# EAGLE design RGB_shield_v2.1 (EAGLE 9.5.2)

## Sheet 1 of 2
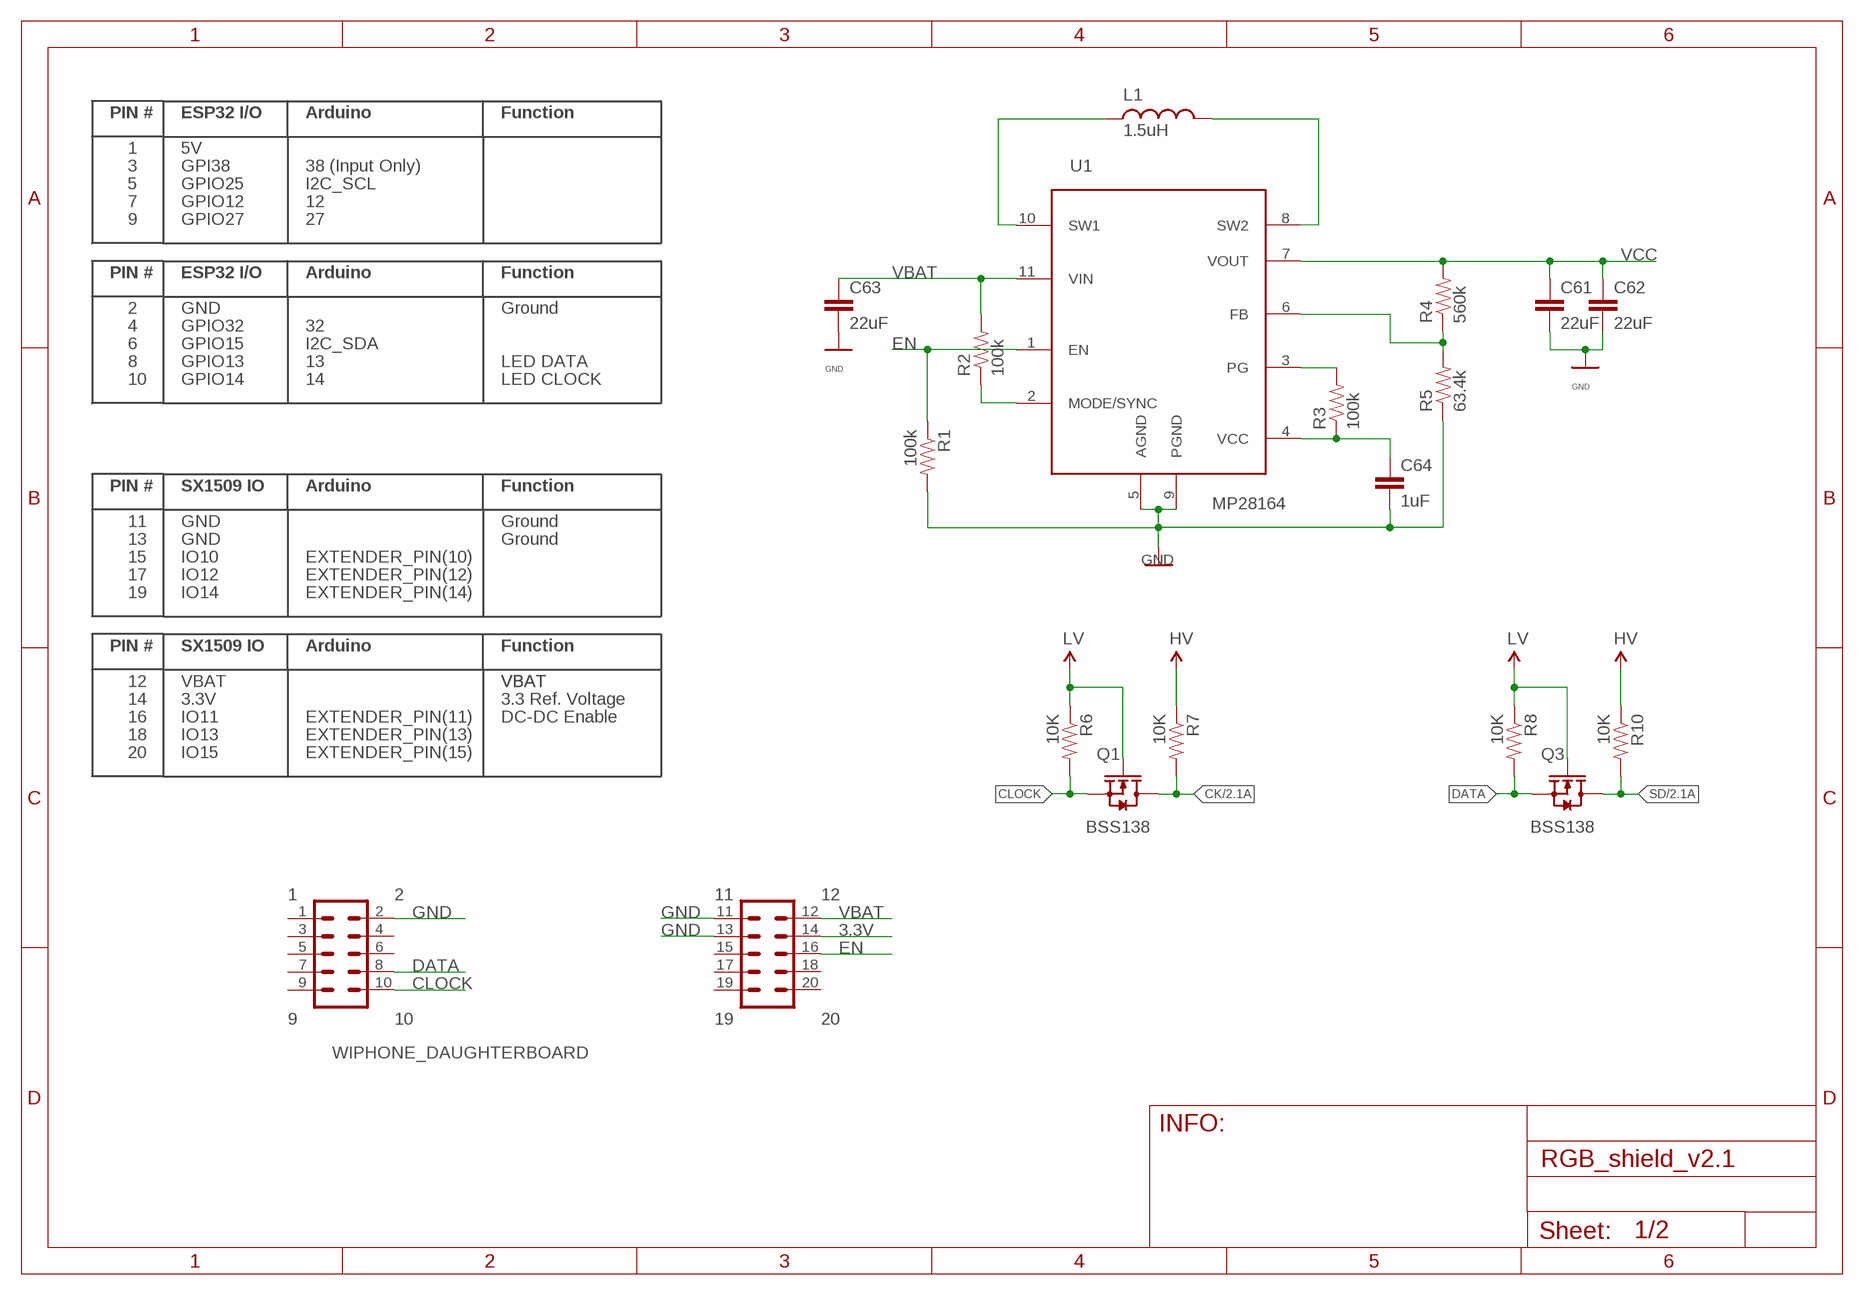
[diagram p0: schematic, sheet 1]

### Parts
C61  22uF  CAP  [0603-CAP-L]
C62  22uF  CAP  [0603-CAP-L]
C63  22uF  CAP0805  [0805_CAP]
C64  1uF  CAP  [0603-CAP-L]
L1  1.5uH  IND0420  [IND04020]
Q1  BSS138  MOSFET_N-L  [SOT23-3-L]
Q3  BSS138  MOSFET_N-L  [SOT23-3-L]
R1  100k  RES  [0603-RES-L]
R2  100k  RES  [0603-RES-L]
R3  100k  RES  [0603-RES-L]
R4  560k  RES  [0603-RES-L]
R5  63.4k  RES  [0603-RES-L]
R6  10K  RES0603  [0603-RES]
R7  10K  RES0603  [0603-RES]
R8  10K  RES0603  [0603-RES]
R10  10K  RES0603  [0603-RES]
U1  MP28164  [QFN11(MP28164)]
WIPHONE_DAUGHTERBOARD-FOOTPRINT1  WIPHONE_DAUGHTERBOARD  [WIPHONE_DAUGHTERBOARD]

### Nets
3.3V: Q1.1(G) Q3.1(G) R6.1 R8.1 WIPHONE_DAUGHTERBOARD-FOOTPRINT1.14 ; supply symbol labelled LV
CK: Q1.3(D) R7.2 ; also sheet 2
CLOCK: Q1.2(S) R6.2 WIPHONE_DAUGHTERBOARD-FOOTPRINT1.10
DATA: Q3.2(S) R8.2 WIPHONE_DAUGHTERBOARD-FOOTPRINT1.8
EN: R1.1 U1.1(EN) WIPHONE_DAUGHTERBOARD-FOOTPRINT1.16
GND: C61.2 C62.2 C63.2 C64.2 R1.2 R5.1 U1.5(AGND) U1.9(PGND) WIPHONE_DAUGHTERBOARD-FOOTPRINT1.2 WIPHONE_DAUGHTERBOARD-FOOTPRINT1.11 WIPHONE_DAUGHTERBOARD-FOOTPRINT1.13 ; also sheet 2
N$157: R2.1 U1.2(MODE/SYNC)
N$158: R3.2 U1.3(PG)
N$159: C64.1 R3.1 U1.4(VCC)
N$162: R4.1 R5.2 U1.6(FB)
SD: Q3.3(D) R10.2 ; also sheet 2
SW1: L1.1 U1.10(SW1)
SW2: L1.2 U1.8(SW2)
VBAT: C63.1 R2.2 U1.11(VIN) WIPHONE_DAUGHTERBOARD-FOOTPRINT1.12
VCC: C61.1 C62.1 R4.2 R7.1 R10.1 U1.7(VOUT) ; supply symbol labelled HV ; also sheet 2
Unconnected: WIPHONE_DAUGHTERBOARD-FOOTPRINT1.3 WIPHONE_DAUGHTERBOARD-FOOTPRINT1.4 WIPHONE_DAUGHTERBOARD-FOOTPRINT1.5 WIPHONE_DAUGHTERBOARD-FOOTPRINT1.6 WIPHONE_DAUGHTERBOARD-FOOTPRINT1.7 WIPHONE_DAUGHTERBOARD-FOOTPRINT1.9 WIPHONE_DAUGHTERBOARD-FOOTPRINT1.15 WIPHONE_DAUGHTERBOARD-FOOTPRINT1.17 WIPHONE_DAUGHTERBOARD-FOOTPRINT1.18 WIPHONE_DAUGHTERBOARD-FOOTPRINT1.19 WIPHONE_DAUGHTERBOARD-FOOTPRINT1.20

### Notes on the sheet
- Ground
- LED DATA
- LED CLOCK
- Ground
- Ground
- VBAT | VBAT
- 3.3 Ref. Voltage
- DC-DC Enable

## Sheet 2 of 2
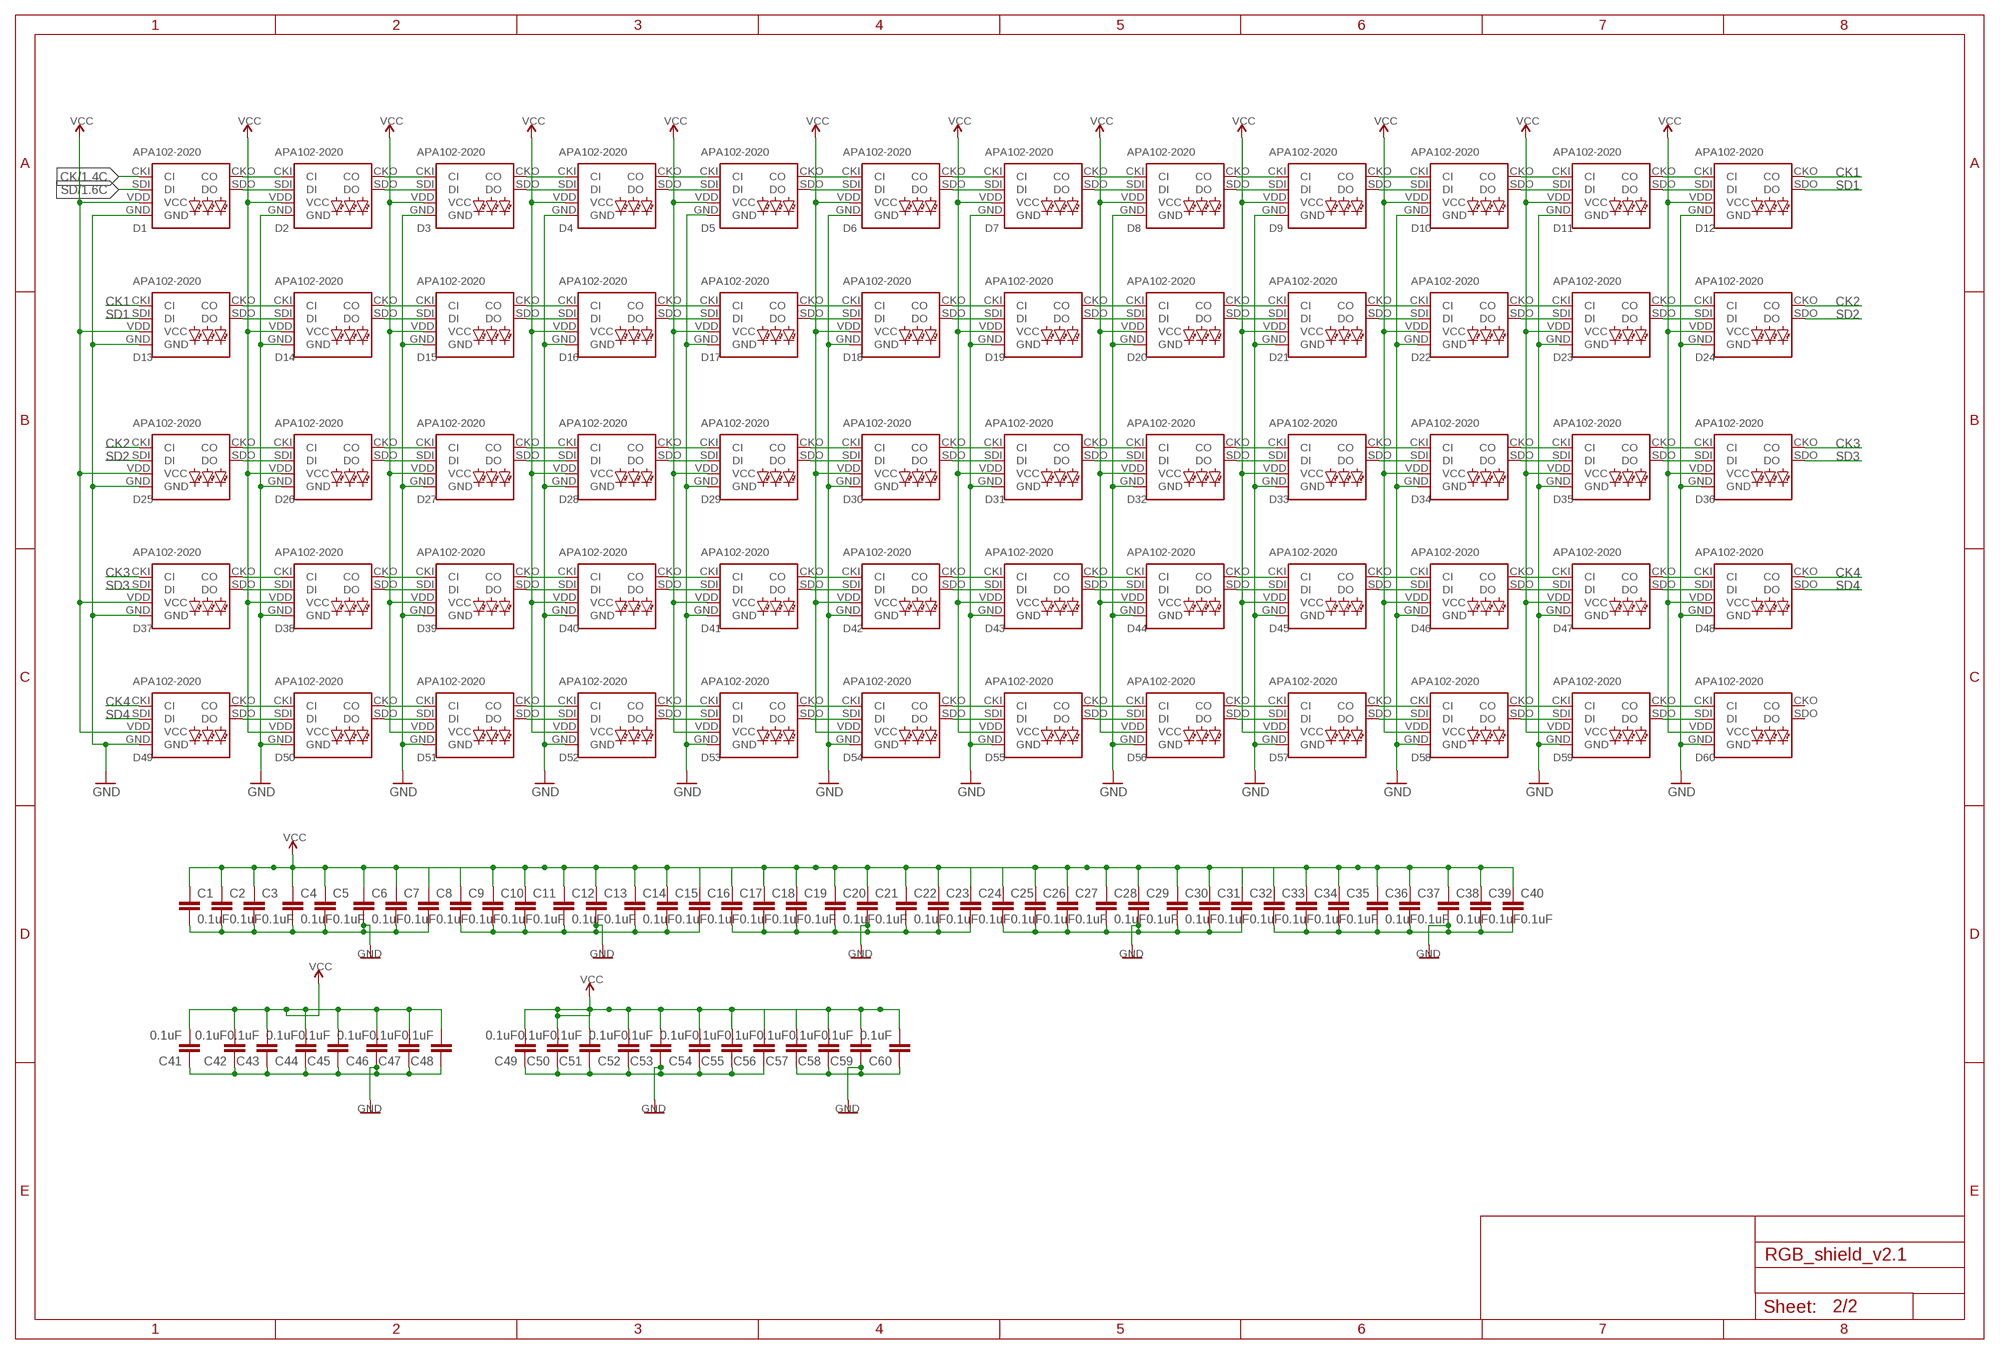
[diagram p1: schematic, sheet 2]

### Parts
C1  0.1uF  CAP0402  [0402-CAP]
C2  0.1uF  CAP0402  [0402-CAP]
C3  0.1uF  CAP0402  [0402-CAP]
C4  0.1uF  CAP0402  [0402-CAP]
C5  0.1uF  CAP0402  [0402-CAP]
C6  0.1uF  CAP0402  [0402-CAP]
C7  0.1uF  CAP0402  [0402-CAP]
C8  0.1uF  CAP0402  [0402-CAP]
C9  0.1uF  CAP0402  [0402-CAP]
C10  0.1uF  CAP0402  [0402-CAP]
C11  0.1uF  CAP0402  [0402-CAP]
C12  0.1uF  CAP0402  [0402-CAP]
C13  0.1uF  CAP0402  [0402-CAP]
C14  0.1uF  CAP0402  [0402-CAP]
C15  0.1uF  CAP0402  [0402-CAP]
C16  0.1uF  CAP0402  [0402-CAP]
C17  0.1uF  CAP0402  [0402-CAP]
C18  0.1uF  CAP0402  [0402-CAP]
C19  0.1uF  CAP0402  [0402-CAP]
C20  0.1uF  CAP0402  [0402-CAP]
C21  0.1uF  CAP0402  [0402-CAP]
C22  0.1uF  CAP0402  [0402-CAP]
C23  0.1uF  CAP0402  [0402-CAP]
C24  0.1uF  CAP0402  [0402-CAP]
C25  0.1uF  CAP0402  [0402-CAP]
C26  0.1uF  CAP0402  [0402-CAP]
C27  0.1uF  CAP0402  [0402-CAP]
C28  0.1uF  CAP0402  [0402-CAP]
C29  0.1uF  CAP0402  [0402-CAP]
C30  0.1uF  CAP0402  [0402-CAP]
C31  0.1uF  CAP0402  [0402-CAP]
C32  0.1uF  CAP0402  [0402-CAP]
C33  0.1uF  CAP0402  [0402-CAP]
C34  0.1uF  CAP0402  [0402-CAP]
C35  0.1uF  CAP0402  [0402-CAP]
C36  0.1uF  CAP0402  [0402-CAP]
C37  0.1uF  CAP0402  [0402-CAP]
C38  0.1uF  CAP0402  [0402-CAP]
C39  0.1uF  CAP0402  [0402-CAP]
C40  0.1uF  CAP0402  [0402-CAP]
C41  0.1uF  CAP0402  [0402-CAP]
C42  0.1uF  CAP0402  [0402-CAP]
C43  0.1uF  CAP0402  [0402-CAP]
C44  0.1uF  CAP0402  [0402-CAP]
C45  0.1uF  CAP0402  [0402-CAP]
C46  0.1uF  CAP0402  [0402-CAP]
C47  0.1uF  CAP0402  [0402-CAP]
C48  0.1uF  CAP0402  [0402-CAP]
C49  0.1uF  CAP0402  [0402-CAP]
C50  0.1uF  CAP0402  [0402-CAP]
C51  0.1uF  CAP0402  [0402-CAP]
C52  0.1uF  CAP0402  [0402-CAP]
C53  0.1uF  CAP0402  [0402-CAP]
C54  0.1uF  CAP0402  [0402-CAP]
C55  0.1uF  CAP0402  [0402-CAP]
C56  0.1uF  CAP0402  [0402-CAP]
C57  0.1uF  CAP0402  [0402-CAP]
C58  0.1uF  CAP0402  [0402-CAP]
C59  0.1uF  CAP0402  [0402-CAP]
C60  0.1uF  CAP0402  [0402-CAP]
D1  APA102-2020  [APA102-2020]
D2  APA102-2020  [APA102-2020]
D3  APA102-2020  [APA102-2020]
D4  APA102-2020  [APA102-2020]
D5  APA102-2020  [APA102-2020]
D6  APA102-2020  [APA102-2020]
D7  APA102-2020  [APA102-2020]
D8  APA102-2020  [APA102-2020]
D9  APA102-2020  [APA102-2020]
D10  APA102-2020  [APA102-2020]
D11  APA102-2020  [APA102-2020]
D12  APA102-2020  [APA102-2020]
D13  APA102-2020  [APA102-2020]
D14  APA102-2020  [APA102-2020]
D15  APA102-2020  [APA102-2020]
D16  APA102-2020  [APA102-2020]
D17  APA102-2020  [APA102-2020]
D18  APA102-2020  [APA102-2020]
D19  APA102-2020  [APA102-2020]
D20  APA102-2020  [APA102-2020]
D21  APA102-2020  [APA102-2020]
D22  APA102-2020  [APA102-2020]
D23  APA102-2020  [APA102-2020]
D24  APA102-2020  [APA102-2020]
D25  APA102-2020  [APA102-2020]
D26  APA102-2020  [APA102-2020]
D27  APA102-2020  [APA102-2020]
D28  APA102-2020  [APA102-2020]
D29  APA102-2020  [APA102-2020]
D30  APA102-2020  [APA102-2020]
D31  APA102-2020  [APA102-2020]
D32  APA102-2020  [APA102-2020]
D33  APA102-2020  [APA102-2020]
D34  APA102-2020  [APA102-2020]
D35  APA102-2020  [APA102-2020]
D36  APA102-2020  [APA102-2020]
D37  APA102-2020  [APA102-2020]
D38  APA102-2020  [APA102-2020]
D39  APA102-2020  [APA102-2020]
D40  APA102-2020  [APA102-2020]
D41  APA102-2020  [APA102-2020]
D42  APA102-2020  [APA102-2020]
D43  APA102-2020  [APA102-2020]
D44  APA102-2020  [APA102-2020]
D45  APA102-2020  [APA102-2020]
D46  APA102-2020  [APA102-2020]
D47  APA102-2020  [APA102-2020]
D48  APA102-2020  [APA102-2020]
D49  APA102-2020  [APA102-2020]
D50  APA102-2020  [APA102-2020]
D51  APA102-2020  [APA102-2020]
D52  APA102-2020  [APA102-2020]
D53  APA102-2020  [APA102-2020]
D54  APA102-2020  [APA102-2020]
D55  APA102-2020  [APA102-2020]
D56  APA102-2020  [APA102-2020]
D57  APA102-2020  [APA102-2020]
D58  APA102-2020  [APA102-2020]
D59  APA102-2020  [APA102-2020]
D60  APA102-2020  [APA102-2020]

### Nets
CK: D1.CKI(CI) ; also sheet 1
CK1: D12.CKO(CO) D13.CKI(CI)
CK2: D24.CKO(CO) D25.CKI(CI)
CK3: D36.CKO(CO) D37.CKI(CI)
CK4: D48.CKO(CO) D49.CKI(CI)
GND: C1.2 C2.2 C3.2 C4.2 C5.2 C6.2 C7.2 C8.2 C9.2 C10.2 C11.2 C12.2 C13.2 C14.2 C15.2 C16.2 C17.2 C18.2 C19.2 C20.2 C21.2 C22.2 C23.2 C24.2 C25.2 C26.2 C27.2 C28.2 C29.2 C30.2 C31.2 C32.2 C33.2 C34.2 C35.2 C36.2 C37.2 C38.2 C39.2 C40.2 C41.1 C42.1 C43.1 C44.1 C45.1 C46.1 C47.1 C48.1 C49.1 C50.1 C51.1 C52.1 C53.1 C54.1 C55.1 C56.1 C57.1 C58.1 C59.1 C60.1 D1.GND D2.GND D3.GND D4.GND D5.GND D6.GND D7.GND D8.GND D9.GND D10.GND D11.GND D12.GND D13.GND D14.GND D15.GND D16.GND D17.GND D18.GND D19.GND D20.GND D21.GND D22.GND D23.GND D24.GND D25.GND D26.GND D27.GND D28.GND D29.GND D30.GND D31.GND D32.GND D33.GND D34.GND D35.GND D36.GND D37.GND D38.GND D39.GND D40.GND D41.GND D42.GND D43.GND D44.GND D45.GND D46.GND D47.GND D48.GND D49.GND D50.GND D51.GND D52.GND D53.GND D54.GND D55.GND D56.GND D57.GND D58.GND D59.GND D60.GND ; also sheet 1
N$1: D1.CKO(CO) D2.CKI(CI)
N$2: D1.SDO(DO) D2.SDI(DI)
N$3: D2.CKO(CO) D3.CKI(CI)
N$4: D2.SDO(DO) D3.SDI(DI)
N$5: D3.CKO(CO) D4.CKI(CI)
N$6: D3.SDO(DO) D4.SDI(DI)
N$7: D4.CKO(CO) D5.CKI(CI)
N$8: D4.SDO(DO) D5.SDI(DI)
N$11: D5.CKO(CO) D6.CKI(CI)
N$12: D5.SDO(DO) D6.SDI(DI)
N$13: D6.CKO(CO) D7.CKI(CI)
N$14: D6.SDO(DO) D7.SDI(DI)
N$15: D7.CKO(CO) D8.CKI(CI)
N$16: D7.SDO(DO) D8.SDI(DI)
N$17: D8.CKO(CO) D9.CKI(CI)
N$18: D8.SDO(DO) D9.SDI(DI)
N$19: D9.CKO(CO) D10.CKI(CI)
N$20: D9.SDO(DO) D10.SDI(DI)
N$21: D10.CKO(CO) D11.CKI(CI)
N$22: D10.SDO(DO) D11.SDI(DI)
N$23: D11.CKO(CO) D12.CKI(CI)
N$24: D11.SDO(DO) D12.SDI(DI)
N$25: D13.CKO(CO) D14.CKI(CI)
N$26: D13.SDO(DO) D14.SDI(DI)
N$27: D14.CKO(CO) D15.CKI(CI)
N$28: D14.SDO(DO) D15.SDI(DI)
N$29: D15.CKO(CO) D16.CKI(CI)
N$30: D15.SDO(DO) D16.SDI(DI)
N$31: D16.CKO(CO) D17.CKI(CI)
N$32: D16.SDO(DO) D17.SDI(DI)
N$33: D17.CKO(CO) D18.CKI(CI)
N$34: D17.SDO(DO) D18.SDI(DI)
N$35: D18.CKO(CO) D19.CKI(CI)
N$36: D18.SDO(DO) D19.SDI(DI)
N$38: D19.CKO(CO) D20.CKI(CI)
N$40: D19.SDO(DO) D20.SDI(DI)
N$42: D20.CKO(CO) D21.CKI(CI)
N$43: D20.SDO(DO) D21.SDI(DI)
N$45: D21.CKO(CO) D22.CKI(CI)
N$47: D21.SDO(DO) D22.SDI(DI)
N$49: D22.CKO(CO) D23.CKI(CI)
N$50: D22.SDO(DO) D23.SDI(DI)
N$51: D23.CKO(CO) D24.CKI(CI)
N$52: D23.SDO(DO) D24.SDI(DI)
N$53: D25.CKO(CO) D26.CKI(CI)
N$54: D25.SDO(DO) D26.SDI(DI)
N$55: D26.CKO(CO) D27.CKI(CI)
N$56: D26.SDO(DO) D27.SDI(DI)
N$57: D27.CKO(CO) D28.CKI(CI)
N$58: D27.SDO(DO) D28.SDI(DI)
N$59: D28.CKO(CO) D29.CKI(CI)
N$60: D28.SDO(DO) D29.SDI(DI)
N$61: D29.CKO(CO) D30.CKI(CI)
N$62: D29.SDO(DO) D30.SDI(DI)
N$63: D30.CKO(CO) D31.CKI(CI)
N$64: D30.SDO(DO) D31.SDI(DI)
N$66: D31.CKO(CO) D32.CKI(CI)
N$67: D31.SDO(DO) D32.SDI(DI)
N$68: D32.CKO(CO) D33.CKI(CI)
N$69: D32.SDO(DO) D33.SDI(DI)
N$70: D33.CKO(CO) D34.CKI(CI)
N$72: D33.SDO(DO) D34.SDI(DI)
N$73: D34.CKO(CO) D35.CKI(CI)
N$74: D34.SDO(DO) D35.SDI(DI)
N$75: D35.CKO(CO) D36.CKI(CI)
N$77: D35.SDO(DO) D36.SDI(DI)
N$79: D37.CKO(CO) D38.CKI(CI)
N$81: D37.SDO(DO) D38.SDI(DI)
N$82: D38.CKO(CO) D39.CKI(CI)
N$91: D38.SDO(DO) D39.SDI(DI)
N$102: D39.CKO(CO) D40.CKI(CI)
N$103: D39.SDO(DO) D40.SDI(DI)
N$104: D40.CKO(CO) D41.CKI(CI)
N$105: D40.SDO(DO) D41.SDI(DI)
N$106: D41.CKO(CO) D42.CKI(CI)
N$107: D41.SDO(DO) D42.SDI(DI)
N$108: D42.CKO(CO) D43.CKI(CI)
N$109: D42.SDO(DO) D43.SDI(DI)
N$110: D43.CKO(CO) D44.CKI(CI)
N$111: D43.SDO(DO) D44.SDI(DI)
N$112: D44.CKO(CO) D45.CKI(CI)
N$113: D44.SDO(DO) D45.SDI(DI)
N$114: D45.CKO(CO) D46.CKI(CI)
N$115: D45.SDO(DO) D46.SDI(DI)
N$116: D46.CKO(CO) D47.CKI(CI)
N$117: D46.SDO(DO) D47.SDI(DI)
N$118: D47.CKO(CO) D48.CKI(CI)
N$119: D47.SDO(DO) D48.SDI(DI)
N$120: D49.CKO(CO) D50.CKI(CI)
N$121: D49.SDO(DO) D50.SDI(DI)
N$122: D50.CKO(CO) D51.CKI(CI)
N$123: D50.SDO(DO) D51.SDI(DI)
N$124: D51.CKO(CO) D52.CKI(CI)
N$125: D51.SDO(DO) D52.SDI(DI)
N$126: D52.CKO(CO) D53.CKI(CI)
N$127: D52.SDO(DO) D53.SDI(DI)
N$128: D53.CKO(CO) D54.CKI(CI)
N$129: D53.SDO(DO) D54.SDI(DI)
N$130: D54.CKO(CO) D55.CKI(CI)
N$131: D54.SDO(DO) D55.SDI(DI)
N$132: D55.CKO(CO) D56.CKI(CI)
N$133: D55.SDO(DO) D56.SDI(DI)
N$134: D57.CKO(CO) D58.CKI(CI)
N$135: D57.SDO(DO) D58.SDI(DI)
N$136: D58.CKO(CO) D59.CKI(CI)
N$137: D58.SDO(DO) D59.SDI(DI)
N$138: D59.CKO(CO) D60.CKI(CI)
N$139: D59.SDO(DO) D60.SDI(DI)
N$140: D56.CKO(CO) D57.CKI(CI)
N$141: D56.SDO(DO) D57.SDI(DI)
SD: D1.SDI(DI) ; also sheet 1
SD1: D12.SDO(DO) D13.SDI(DI)
SD2: D24.SDO(DO) D25.SDI(DI)
SD3: D36.SDO(DO) D37.SDI(DI)
SD4: D48.SDO(DO) D49.SDI(DI)
VCC: C1.1 C2.1 C3.1 C4.1 C5.1 C6.1 C7.1 C8.1 C9.1 C10.1 C11.1 C12.1 C13.1 C14.1 C15.1 C16.1 C17.1 C18.1 C19.1 C20.1 C21.1 C22.1 C23.1 C24.1 C25.1 C26.1 C27.1 C28.1 C29.1 C30.1 C31.1 C32.1 C33.1 C34.1 C35.1 C36.1 C37.1 C38.1 C39.1 C40.1 C41.2 C42.2 C43.2 C44.2 C45.2 C46.2 C47.2 C48.2 C49.2 C50.2 C51.2 C52.2 C53.2 C54.2 C55.2 C56.2 C57.2 C58.2 C59.2 C60.2 D1.VDD(VCC) D2.VDD(VCC) D3.VDD(VCC) D4.VDD(VCC) D5.VDD(VCC) D6.VDD(VCC) D7.VDD(VCC) D8.VDD(VCC) D9.VDD(VCC) D10.VDD(VCC) D11.VDD(VCC) D12.VDD(VCC) D13.VDD(VCC) D14.VDD(VCC) D15.VDD(VCC) D16.VDD(VCC) D17.VDD(VCC) D18.VDD(VCC) D19.VDD(VCC) D20.VDD(VCC) D21.VDD(VCC) D22.VDD(VCC) D23.VDD(VCC) D24.VDD(VCC) D25.VDD(VCC) D26.VDD(VCC) D27.VDD(VCC) D28.VDD(VCC) D29.VDD(VCC) D30.VDD(VCC) D31.VDD(VCC) D32.VDD(VCC) D33.VDD(VCC) D34.VDD(VCC) D35.VDD(VCC) D36.VDD(VCC) D37.VDD(VCC) D38.VDD(VCC) D39.VDD(VCC) D40.VDD(VCC) D41.VDD(VCC) D42.VDD(VCC) D43.VDD(VCC) D44.VDD(VCC) D45.VDD(VCC) D46.VDD(VCC) D47.VDD(VCC) D48.VDD(VCC) D49.VDD(VCC) D50.VDD(VCC) D51.VDD(VCC) D52.VDD(VCC) D53.VDD(VCC) D54.VDD(VCC) D55.VDD(VCC) D56.VDD(VCC) D57.VDD(VCC) D58.VDD(VCC) D59.VDD(VCC) D60.VDD(VCC) ; also sheet 1
Unconnected: D60.CKO(CO) D60.SDO(DO)

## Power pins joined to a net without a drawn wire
1: WIPHONE_DAUGHTERBOARD-FOOTPRINT1.1

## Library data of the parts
C1-C64 = WiPhone:CAP: Capacitor.
D1-D60 = WiPhone:APA102: APA102 Addressable RGB LED Used in manufacturing of various products at SparkFun Packages: 5050 2020 SparkFun Products: SparkFun Lumenati Boards; PROD_ID: DIO-13883
L1 = WiPhone:IND: Inductor.
Q1 Q3 = WiPhone:MOSFET_N: N-Channel Mosfet
R1-R8 R10 = WiPhone:RES: Resistor.
U1 = WiPhone:MP28164
WIPHONE_DAUGHTERBOARD-FOOTPRINT1 = WiPhone:WIPHONE_DAUGHTERBOARD

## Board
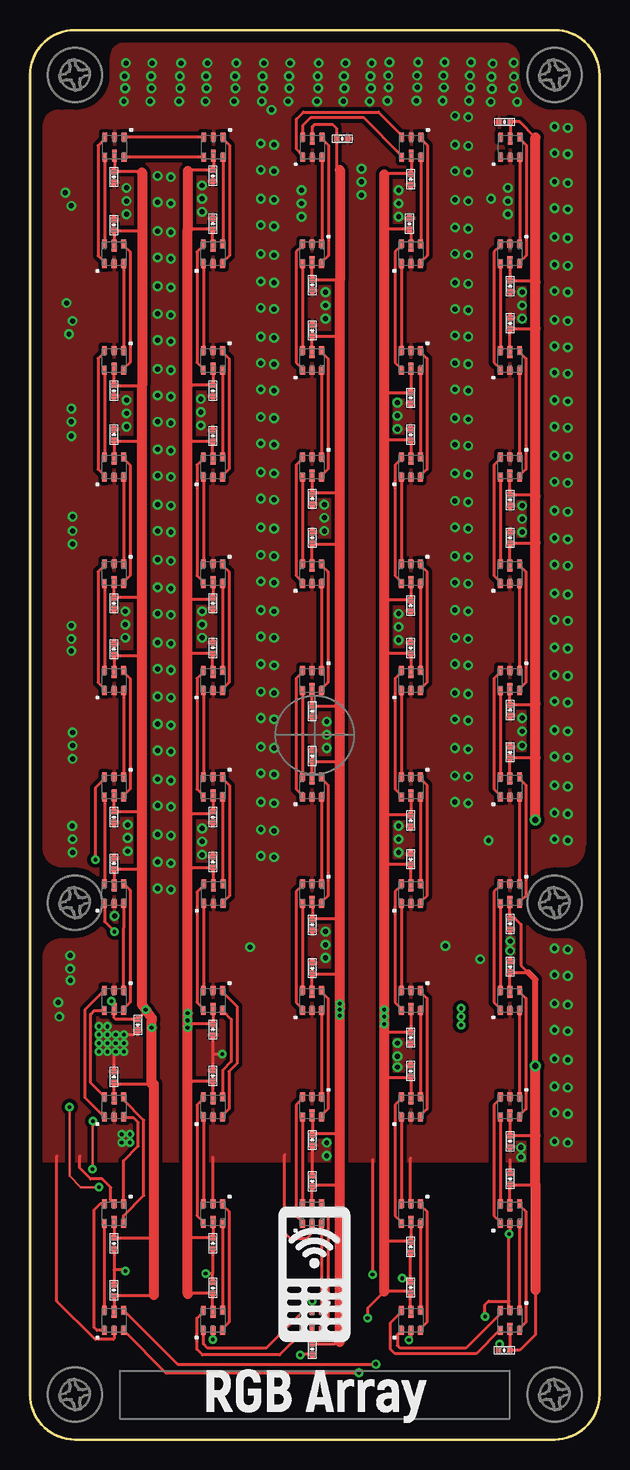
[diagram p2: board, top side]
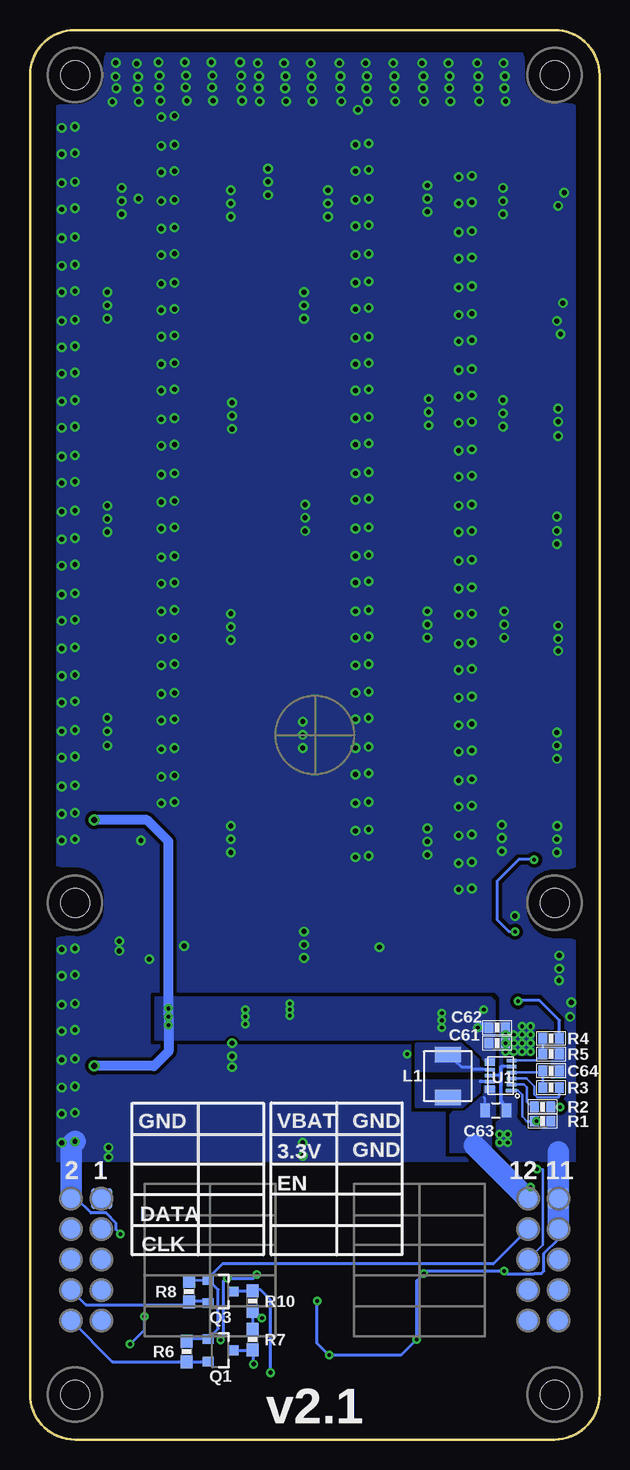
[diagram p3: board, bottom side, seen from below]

Size 47.5 x 117.5 mm. Coordinates in mm from the lower left corner, seen from the top.
Copper layers (1*16): Top 0.035mm / dielectric 1.5mm / Bottom 0.035mm
Design rules "2LDaughterBoards *": minimum track width 6mil, minimum drill 0.3mm, track to track 8mil, track to pad 8mil, pad to pad 8mil, via to via 8mil, smd to smd 0mil, copper to edge 16mil, drill to drill 6mil, minimum pad ring 10mil, minimum via ring 8mil, stop-mask expansion 4mil, vias tented up to drill 25mil, thermal gap 10mil

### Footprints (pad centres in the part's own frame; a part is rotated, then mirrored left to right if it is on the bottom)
0402-CAP = smd 0.508 x 0.508: 1 -0.457,0; 2 0.457,0
0603-CAP-L = smd 0.75 x 0.9: 1 -0.7,0; 2 0.7,0
0805_CAP = smd 0.8 x 1.2: 1 -0.9,0; 2 0.9,0
APA102-2020 = smd 0.4 x 0.7: CKI -0.8,-0.85; CKO 0.8,-0.85; GND 0,0.85; SDI -0.8,0.85; SDO 0.8,0.85 | smd 0.4 x 1: VDD 0,-0.7
IND04020 = smd 1.295 x 2.184: 1 -1.85,0; 2 1.748,0
SOT23-3-L = smd 0.8 x 0.9: 1 -0.95,-1; 2 0.95,-1; 3 0,1.1
0603-RES-L = smd 0.75 x 0.9: 1 -0.7,0; 2 0.7,0
0603-RES = smd 1.1 x 1: 1 -0.85,0; 2 0.85,0
QFN11(MP28164) = smd 0.9 x 0.3: 1 -0.9,1.25 | smd 0.8 x 0.3: 2 -0.9,0.75; 3 -0.9,0.25; 4 -0.9,-0.25; 5 -0.9,-0.75; 6 -0.9,-1.25; 8 0.9,-0.5; 9 0.9,0; 10 0.9,0.5 | smd 0.8 x 0.6: 7 0.9,-1.125; 11 0.9,1.125
WIPHONE_DAUGHTERBOARD = smd 1.75 x 1.75 bottom: 1 17.78,-38.66; 2 20.32,-38.66; 3 17.78,-41.2; 4 20.32,-41.2; 5 17.78,-43.74; 6 20.32,-43.74; 7 17.78,-46.28; 8 20.32,-46.28; 9 17.78,-48.82; 10 20.32,-48.82; 11 -20.32,-38.66; 12 -17.78,-38.66; 13 -20.32,-41.2; 14 -17.78,-41.2; 15 -20.32,-43.74; 16 -17.78,-43.74; 17 -20.32,-46.28; 18 -17.78,-46.28; 19 -20.32,-48.82; 20 -17.78,-48.82 | hole 2.4: 20,-54.991; -20,-54.991; 20,-13.991; 20,55.009; -20,55.009; -20,-13.991

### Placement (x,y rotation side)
C1  39.59,109.84 180 top
C2  40.05,96.14 270 top
C3  40.05,93.05 90 top
C4  40.05,78.32 270 top
C5  40.05,75.17 90 top
C6  40.05,60.8 270 top
C7  40.05,57.29 90 top
C8  40.05,42.98 270 top
C9  40.05,39.41 90 top
C10  40.05,24.86 270 top
C11  40.05,21.73 90 top
C12  39.55,7.44 180 top
C13  31.75,12.67 90 top
C14  31.75,16.05 270 top
C15  31.75,30.72 90 top
C16  31.75,33.5 270 top
C17  31.75,48.37 90 top
C18  31.75,51.59 270 top
C19  31.75,65.98 90 top
C20  31.75,69.51 270 top
C21  31.75,83.76 90 top
C22  31.75,86.83 270 top
C23  31.65,101.34 90 top
C24  31.75,105.05 270 top
C25  26.04,108.44 0 top
C26  23.55,96.24 270 top
C27  23.55,92.45 90 top
C28  23.55,78.42 270 top
C29  23.55,75.17 90 top
C30  23.55,60.7 270 top
C31  23.55,56.99 90 top
C32  23.55,42.91 270 top
C33  23.55,39.28 90 top
C34  23.55,24.96 270 top
C35  23.55,21.53 90 top
C36  23.55,7.54 270 top
C37  15.25,12.64 90 top
C38  15.25,16.35 270 top
C39  15.25,30.32 90 top
C40  15.25,34.17 270 top
C41  15.25,48.14 270 top
C42  15.25,51.89 90 top
C43  15.25,65.98 270 top
C44  15.25,69.71 90 top
C45  15.25,83.66 270 top
C46  15.25,87.43 90 top
C47  15.25,101.34 270 top
C48  15.25,105.35 90 top
C49  7.01,105.25 90 top
C50  7.01,101.24 270 top
C51  7.01,87.43 90 top
C52  7.01,83.76 270 top
C53  7.01,69.71 90 top
C54  7.01,65.88 270 top
C55  7.01,51.89 90 top
C56  7.01,48 270 top
C57  9,34.57 90 top
C58  7.01,30.22 270 top
C59  7.01,16.35 90 top
C60  7.01,12.44 270 top
C61  8.55,33.04 0 bottom
C62  8.55,34.34 0 bottom
C63  8.65,27.44 0 bottom
C64  4.05,30.74 0 bottom
D1  7.01,9.94 180 top
D2  7.01,18.83 0 top
D3  7.01,27.72 180 top
D4  7.01,36.61 0 top
D5  7.01,45.5 180 top
D6  7.01,54.39 0 top
D7  7.01,63.28 180 top
D8  7.01,72.17 0 top
D9  7.01,81.06 180 top
D10  7.01,89.95 0 top
D11  7.01,98.84 180 top
D12  7.05,107.74 0 top
D13  15.3,107.74 0 top
D14  15.26,98.84 180 top
D15  15.26,89.95 0 top
D16  15.26,81.06 180 top
D17  15.26,72.17 0 top
D18  15.26,63.28 180 top
D19  15.26,54.39 0 top
D20  15.3,45.5 180 top
D21  15.26,36.61 0 top
D22  15.26,27.72 180 top
D23  15.26,18.83 0 top
D24  15.26,9.94 180 top
D25  23.52,9.94 0 top
D26  23.52,18.83 180 top
D27  23.52,27.72 0 top
D28  23.52,36.61 180 top
D29  23.52,45.5 0 top
D30  23.52,54.39 180 top
D31  23.52,63.28 0 top
D32  23.52,72.17 180 top
D33  23.52,81.06 0 top
D34  23.52,89.95 180 top
D35  23.52,98.84 0 top
D36  23.55,107.74 180 top
D37  31.8,107.74 0 top
D38  31.77,98.84 180 top
D39  31.77,89.95 0 top
D40  31.77,81.06 180 top
D41  31.77,72.17 0 top
D42  31.77,63.28 180 top
D43  31.77,54.39 0 top
D44  31.77,45.5 180 top
D45  31.77,36.61 0 top
D46  31.77,27.72 180 top
D47  31.77,18.83 0 top
D48  31.77,9.94 180 top
D49  40.03,9.94 0 top
D50  40.03,18.83 180 top
D51  40.03,27.72 0 top
D52  40.03,36.61 180 top
D53  40.03,45.5 0 top
D54  40.03,54.39 180 top
D55  40.03,63.28 0 top
D56  40.03,72.17 180 top
D57  40.03,81.06 0 top
D58  40.03,89.95 180 top
D59  40.03,98.84 0 top
D60  40.05,107.74 180 top
L1  12.65,30.34 90 bottom
Q1  31.65,7.44 270 bottom
Q3  31.65,12.34 270 bottom
R1  4.75,26.54 0 bottom
R2  4.75,27.74 0 bottom
R3  4.05,29.34 0 bottom
R4  4.05,33.44 0 bottom
R5  4.05,32.14 180 bottom
R6  34.45,7.34 270 bottom
R7  28.95,8.34 270 bottom
R8  34.25,12.34 270 bottom
R10  28.95,11.54 90 bottom
U1  8.25,30.34 180 bottom
WIPHONE_DAUGHTERBOARD-FOOTPRINT1  23.75,58.74 0 top

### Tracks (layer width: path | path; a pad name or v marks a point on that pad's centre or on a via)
3.3V
  Bottom 0.203: Q3.1 32.75,13.29 34.15,13.29
  Bottom 0.254: R6.1 34.25,8.39 Q1.1 31.81,9.23 31.81,12.5 32.6,13.29 32.75,13.29 | WIPHONE_DAUGHTERBOARD-FOOTPRINT1.14 8.87,14.64 31.45,14.64 32.65,13.44 Q3.1
  Bottom 0.305: 34.15,13.29 R8.1
CK  (via drill 0.35)
  Top 0.254: D1.CKI 12.32,6.28 v28.84,6.28
  Bottom 0.254: Q1.3 29,7.44 | 29,7.44 R7.2 | v28.84,6.28 28.84,7.28 29,7.44
CK1
  Top 0.254: D13.CKI D12.CKO
CK2
  Top 0.254: D25.CKI 22.72,8.94 20.83,7.05 14.38,7.05 13.93,7.5 13.93,10.11 14.46,10.64 D24.CKO
CK3
  Top 0.254: D37.CKI 31,107.04 27.87,110.17 23.4,110.17 22.75,109.52 D36.CKO
CK4
  Top 0.254: D49.CKI 39.17,9.09 37.23,7.15 30.45,7.15 30.08,7.52 30.08,9.75 30.97,10.64 D48.CKO
CLOCK
  Bottom 0.254: WIPHONE_DAUGHTERBOARD-FOOTPRINT1.10 40.64,6.49 R6.2 Q1.2
DATA
  Bottom 0.254: WIPHONE_DAUGHTERBOARD-FOOTPRINT1.8 42.85,11.24 34.5,11.24 34.22,11.52 32.77,11.52 Q3.2
  Bottom 0.305: 34.22,11.52 R8.2
EN  (via drill 0.3)
  Top 0.203: v5.21,22.54 5.21,26.1 5.35,26.24 5.35,26.45 v5.25,26.54
  Bottom 0.203: U1.1 6.8,29.09 6.46,28.75 6.46,26.95 6.05,26.54 v5.25,26.54 R1.1 | WIPHONE_DAUGHTERBOARD-FOOTPRINT1.16 4.75,16.22 4.75,22.54 v5.21,22.54
GND  (via drill 0.3, 0.41)
  Top 0.254: D1.GND 7.01,8.4 6.95,8.34 5.45,8.34 2.25,11.54 2.25,23.64 | D2.GND 6.74,19.95 6.74,21.02 6.03,21.72 5.06,21.72 4.15,22.63 4.15,23.64 | v7.95,14.04 7.85,14.14 7.01,14.14 | v14.65,13.84 15.25,13.84 | D24.GND 15.26,8.36 v15.25,8.34 | v22.55,7.04 22.59,7.08 C36.2 | v23.55,11.54 23.55,10.82 D25.GND | D50.GND 40.03,17.22 v39.95,17.14 39.95,11.54 | D23.GND 15.26,23.56 | D47.GND 31.75,19.71 31.75,23.44 | D49.GND 39.95,10.87 39.95,11.54 | D48.GND 31.77,8.47 v31.6,8.3 | v31.05,13.44 31.43,13.44 C13.2 C14.2 | v37.95,10.24 37.95,11.24 38.25,11.54 39.95,11.54 | D26.GND 23.52,17.21 23.05,16.74 21.75,16.74 21.25,17.24 21.25,23.74 | 28.56,23.34 v28.56,13.74 | C35.2 C34.2 | C40.2 15.25,32.14 | 15.25,32.14 C39.2 | 15.25,32.14 v16.05,32.14 | C11.2 40.05,23.34 | v39.15,7.94 39.15,7.5 C12.2 | C38.2 15.25,13.84 | C37.2 15.25,13.84 | C59.1 7.01,14.14 | 7.01,14.14 C60.1 | C57.1 8.63,33.74 v7.85,33.74 | C58.1 7.01,32.2 v7.15,32.34
  Bottom 0.254: U1.5 8.2,31.09 | 8.25,30.34 U1.9 | WIPHONE_DAUGHTERBOARD-FOOTPRINT1.13 3.43,16.71 4.63,15.5 4.63,14.06 4.85,13.84 5.42,13.84 5.47,13.8 7.7,13.8 v7.95,14.04 14.45,14.04 v14.65,13.84 15.25,13.24 v15.25,8.34 16.55,7.04 v22.55,7.04 23.55,8.04 v23.55,11.54 | v39.95,17.14 40.32,17.52 40.32,18.04 41.16,18.88 42.41,18.88 43.62,20.08 WIPHONE_DAUGHTERBOARD-FOOTPRINT1.2 | v31.6,8.3 31.35,8.55 31.35,13.24 31.15,13.44 v31.05,13.44 28.86,13.44 v28.56,13.74 | v39.15,7.94 37.95,9.14 v37.95,10.24
  Bottom 0.305: 8.2,31.09 8.25,31.04 8.25,30.34 8.25,28.24 C63.2
  Bottom 1.778: WIPHONE_DAUGHTERBOARD-FOOTPRINT1.13 WIPHONE_DAUGHTERBOARD-FOOTPRINT1.11 3.43,23.96 | WIPHONE_DAUGHTERBOARD-FOOTPRINT1.2 44.07,24.52 v43.75,24.84
  other vias: 38.25,49.94 38.45,103.44 34.65,41.14 20.15,110.84 3.45,102.84 3.55,93.24 3.45,84.84 3.55,75.74 3.45,66.74 3.55,57.84 3.55,48.94 3.35,40.34 18.35,41.04 2.45,35.24 43.75,27.24 43.75,31.74 43.75,29.44 43.75,34.14 43.75,36.34 43.75,38.74 43.75,40.94 43.75,54.54 43.75,52.24 43.75,50.04 43.75,56.94 43.75,59.14 43.75,61.54 43.75,77.44 43.75,75.14 43.75,68.34 43.75,70.54 43.75,72.94 43.75,66.04 43.75,63.74 43.75,79.84 43.75,82.04 43.75,84.44 43.75,91.14 43.75,93.34 43.75,95.74 43.75,88.94 43.75,86.64 43.75,100.24 43.75,97.94 43.75,102.64 43.75,104.84 43.75,107.24 43.75,109.44 44.85,24.74 44.85,27.14 44.85,31.64 44.85,29.34 44.85,34.04 44.85,36.24 44.85,38.64 44.85,40.84 44.85,54.44 44.85,52.14 44.85,49.94 44.85,56.84 44.85,59.04 44.85,61.44 44.85,77.34 44.85,75.04 44.85,68.24 44.85,70.44 44.85,72.84 44.85,65.94 44.85,63.64 44.85,79.74 44.85,81.94 44.85,84.34 44.85,91.04 44.85,93.24 44.85,95.64 44.85,88.84 44.85,86.54 44.85,100.14 44.85,97.84 44.85,102.54 44.85,104.74 44.85,107.14 44.85,109.34 2.95,103.94 3.05,94.74 3.25,92.14 3.45,85.94 3.45,83.64 3.55,76.94 3.55,74.64 3.45,65.74 3.45,67.84 3.55,58.94 3.55,56.74 3.55,50.04 3.53,51.14 3.37,38.27 3.35,39.24 2.35,36.44 8.35,24.74 8.35,25.44 7.65,24.74 7.65,25.44 7.85,32.34 7.85,33.04 7.15,33.04 7.15,33.74 6.45,32.34 6.45,33.04 6.45,33.74 6.45,34.44 5.75,32.34 5.75,33.04 5.75,33.74 5.75,34.44 8.05,103.24 8.05,104.34 8.05,102.14 14.35,103.44 14.35,104.54 14.35,102.34 8.05,85.54 8.05,86.64 8.05,84.44 14.25,85.64 14.25,86.74 14.25,84.54 7.95,67.94 7.95,69.04 7.95,66.84 14.35,67.94 14.35,69.04 14.35,66.84 8.15,50.14 8.15,51.24 8.15,49.04 14.35,49.84 14.35,50.94 14.35,48.74 22.65,103.04 22.65,104.14 22.65,101.94 39.85,103.24 39.85,104.34 39.85,102.14 30.75,103.04 30.75,104.14 30.75,101.94 41.05,94.54 41.05,95.64 41.05,93.44 24.65,94.54 24.65,95.64 24.65,93.44 30.65,85.34 30.65,86.44 30.65,84.24 24.55,76.84 24.55,77.94 24.55,75.74 41.05,76.74 41.05,77.84 41.05,75.64 30.75,67.74 30.75,68.84 30.75,66.64 24.75,58.74 24.75,59.84 24.75,57.64 41.05,59.04 41.05,60.14 41.05,57.84 30.75,50.04 30.75,51.14 30.75,48.94 24.65,41.24 24.65,42.34 24.65,40.14 24.75,23.64 24.75,24.74 30.65,31.94 30.65,33.04 30.65,31.04 40.95,24.34 40.95,23.54 27.65,104.84 27.65,105.94 27.65,103.74 40.05,40.74 40.05,41.54 37.55,40.04 19.25,53.14 19.25,50.84 19.25,48.64 19.25,55.54 19.25,57.74 19.25,60.14 19.25,76.04 19.25,73.74 19.25,66.94 19.25,69.14 19.25,71.54 19.25,64.64 19.25,62.34 19.25,78.44 19.25,80.64 19.25,83.04 19.25,89.74 19.25,91.94 19.25,94.34 19.25,87.54 19.25,85.24 19.25,98.84 19.25,96.54 19.25,101.24 19.25,103.44 19.25,105.84 19.25,108.04 20.35,53.04 20.35,50.74 20.35,48.54 20.35,55.44 20.35,57.64 20.35,60.04 20.35,75.94 20.35,73.64 20.35,66.84 20.35,69.04 20.35,71.44 20.35,64.54 20.35,62.24 20.35,78.34 20.35,80.54 20.35,82.94 20.35,89.64 20.35,91.84 20.35,94.24 20.35,87.44 20.35,85.14 20.35,98.74 20.35,96.44 20.35,101.14 20.35,103.34 20.35,105.74 20.35,107.94 35.45,57.64 35.45,55.34 35.45,53.14 35.45,60.04 35.45,62.24 35.45,64.64 35.45,80.54 35.45,78.24 35.45,71.44 35.45,73.64 35.45,76.04 35.45,69.14 35.45,66.84 35.45,82.94 35.45,85.14 35.45,87.54 35.45,94.24 35.45,96.44 35.45,98.84 35.45,92.04 35.45,89.74 35.45,103.34 35.45,101.04 35.45,105.74 35.45,107.94 35.45,110.34 36.55,57.54 36.55,55.24 36.55,53.04 36.55,59.94 36.55,62.14 36.55,64.54 36.55,80.44 36.55,78.14 36.55,71.34 36.55,73.54 36.55,75.94 36.55,69.04 36.55,66.74 36.55,82.84 36.55,85.04 36.55,87.44 36.55,94.14 36.55,96.34 36.55,98.74 36.55,91.94 36.55,89.64 36.55,103.24 36.55,100.94 36.55,105.64 36.55,107.84 36.55,110.24 10.65,50.44 10.65,48.14 10.65,45.94 10.65,52.84 10.65,55.04 10.65,57.44 10.65,73.34 10.65,71.04 10.65,64.24 10.65,66.44 10.65,68.84 10.65,61.94 10.65,59.64 10.65,75.74 10.65,77.94 10.65,80.34 10.65,87.04 10.65,89.24 10.65,91.64 10.65,84.84 10.65,82.54 10.65,96.14 10.65,93.84 10.65,98.54 10.65,100.74 10.65,103.14 10.65,105.34 11.75,50.34 11.75,48.04 11.75,45.84 11.75,52.74 11.75,54.94 11.75,57.34 11.75,73.24 11.75,70.94 11.75,64.14 11.75,66.34 11.75,68.74 11.75,61.84 11.75,59.54 11.75,75.64 11.75,77.84 11.75,80.24 11.75,86.94 11.75,89.14 11.75,91.54 11.75,84.74 11.75,82.44 11.75,96.04 11.75,93.74 11.75,98.44 11.75,100.64 11.75,103.04 11.75,105.24 7.05,43.64 26.13,111.55 23.93,111.55 21.53,111.55 28.33,111.55 17.03,111.55 19.33,111.55 14.63,111.55 12.43,111.55 10.03,111.55 7.83,111.55 26.23,112.65 24.03,112.65 21.63,112.65 28.43,112.65 17.13,112.65 19.43,112.65 14.73,112.65 12.53,112.65 10.13,112.65 7.93,112.65 26.2,113.64 24,113.64 21.6,113.64 28.4,113.64 17.1,113.64 19.4,113.64 14.7,113.64 12.5,113.64 10.1,113.64 7.9,113.64 26.3,114.74 24.09,114.74 21.7,114.74 28.5,114.74 17.21,114.74 19.51,114.74 14.8,114.74 12.61,114.74 10.2,114.74 8.01,114.74 34.48,113.7 32.28,113.7 29.88,113.7 36.68,113.7 34.59,114.81 32.37,114.81 29.99,114.81 36.78,114.81 34.42,111.61 32.22,111.61 29.82,111.61 36.62,111.61 34.52,112.71 32.32,112.71 29.92,112.71 36.72,112.71 38.49,113.6 40.37,113.62 38.59,114.7 40.34,114.76 38.42,111.51 40.62,111.51 38.52,112.61 40.3,112.65
  pour Bottom (isolate 0.305, rank 3, no thermals): 3.84,-0.1 arc-90 -0.01,3.75 -0.01,113.75 arc-90 3.84,117.6 43.84,117.6 arc-90 47.69,113.75 47.69,3.75 arc-90 43.84,-0.1
  pour Top (isolate 0.305): 3.84,-0.3 arc-90 -0.01,3.55 -0.01,113.55 arc-90 3.84,117.4 43.84,117.4 arc-90 47.69,113.55 47.69,3.55 arc-90 43.84,-0.3
  cutout Bottom: 0.05,23.04 47.45,23.04 47.45,3.94 arc-90 43.45,-0.06 4.05,-0.06 arc-90 0.05,3.94
  cutout Top: 0.05,23.04 47.45,23.04 47.45,3.94 arc-90 43.45,-0.06 4.05,-0.06 arc-90 0.05,3.94
N$1
  Top 0.254: D1.CKO D2.CKI
N$2
  Top 0.254: D1.SDO 5.6,9.09 5.35,9.34 5.35,19.14 5.89,19.68 D2.SDI
N$3
  Top 0.254: D2.CKO 7.81,18.66 9.49,20.35 9.49,26.61 7.81,28.29 D3.CKI
N$4
  Top 0.254: D3.SDI 7.86,26.82 8.63,26.82 9.03,26.42 9.03,24.46 7.81,23.24 D2.SDO
N$5
  Top 0.254: D3.CKO 5.05,29.73 5.05,35.44 5.37,35.76 D4.CKI
N$6
  Top 0.254: D3.SDO 4.59,28.49 4.59,35.84 D4.SDI
N$7
  Top 0.254: D5.CKI 8.35,45.81 8.35,36.45 7.81,35.91 D4.CKO
N$8
  Top 0.254: D4.SDO 7.81,42.64 7.83,42.66 7.83,44.63 D5.SDI
N$11
  Top 0.254: D6.CKI D5.CKO
N$12  (via drill 0.3)
  Top 0.254: D6.SDI 6.21,55.09 5.45,54.33 v5.45,48.34 | D5.SDO 6.21,43.18 v7.05,42.34
  Bottom 0.254: v5.45,48.34 6.75,48.34 8.55,46.54 8.55,43.34 7.55,42.34 v7.05,42.34
N$13
  Top 0.254: D7.CKI 7.81,63.98 8.34,63.45 8.34,54.22 7.81,53.69 D6.CKO
N$14
  Top 0.254: D7.SDI D6.SDO
N$15
  Top 0.254: D8.CKI D7.CKO
N$16
  Top 0.254: D8.SDI 6.21,72.87 5.68,72.34 5.68,63.11 6.21,62.58 D7.SDO
N$17
  Top 0.254: D9.CKI 7.81,81.76 8.34,81.23 8.34,72 7.81,71.47 D8.CKO
N$18
  Top 0.254: D9.SDI D8.SDO
N$19
  Top 0.254: D10.CKI D9.CKO
N$20
  Top 0.254: D10.SDI 6.21,90.65 5.68,90.12 5.68,80.89 6.21,80.36 D9.SDO
N$21
  Top 0.254: D11.CKI 7.81,99.54 8.34,99.01 8.34,89.78 7.81,89.25 D10.CKO
N$22
  Top 0.254: D11.SDI D10.SDO
N$23
  Top 0.254: D12.CKI 6.25,99.73 D11.CKO
N$24
  Top 0.254: D12.SDI 6.25,108.44 5.68,107.87 5.68,98.67 6.21,98.14 D11.SDO
N$25
  Top 0.254: D13.CKO 16.1,99.73 D14.CKI
N$26
  Top 0.254: D13.SDO 16.1,108.44 16.63,107.91 16.63,98.71 16.06,98.14 D14.SDI
N$27
  Top 0.254: D14.CKO 14.46,99.54 13.93,99.01 13.93,89.78 14.46,89.25 D15.CKI
N$28
  Top 0.254: D14.SDO D15.SDI
N$29
  Top 0.254: D15.CKO D16.CKI
N$30
  Top 0.254: D15.SDO 16.06,90.65 16.59,90.12 16.59,80.89 16.06,80.36 D16.SDI
N$31
  Top 0.254: D16.CKO 14.46,81.76 13.93,81.23 13.93,72 14.46,71.47 D17.CKI
N$32
  Top 0.254: D16.SDO D17.SDI
N$33
  Top 0.254: D17.CKO D18.CKI
N$34
  Top 0.254: D17.SDO 16.06,72.87 16.59,72.34 16.59,63.11 16.06,62.58 D18.SDI
N$35
  Top 0.254: D18.CKO 14.46,63.98 13.93,63.45 13.93,54.22 14.46,53.69 D19.CKI
N$36
  Top 0.254: D18.SDO D19.SDI
N$38
  Top 0.254: D19.CKO 16.06,46.39 D20.CKI
N$40
  Top 0.254: D19.SDO 16.06,55.09 16.63,54.53 16.63,45.33 16.1,44.8 D20.SDI
N$42
  Top 0.254: D20.CKO 14.5,46.2 13.93,45.64 13.93,36.44 14.46,35.91 D21.CKI
N$43
  Top 0.254: D20.SDO 14.5,37.5 D21.SDI
N$45
  Top 0.254: D21.CKO 16.79,35.04 16.79,31.51 16.06,30.78 D22.CKI
N$47
  Top 0.254: D21.SDO 16.06,37.31 17.27,36.11 17.27,31.34 16.59,30.67 16.59,27.55 16.06,27.02 D22.SDI
N$49
  Top 0.254: D22.CKO 14.46,28.42 13.93,27.89 13.93,18.66 14.46,18.13 D23.CKI
N$50
  Top 0.254: D22.SDO D23.SDI
N$51
  Top 0.254: D23.CKO D24.CKI
N$52
  Top 0.254: D23.SDO 16.06,19.53 16.59,19 16.59,9.77 16.06,9.24 D24.SDI
N$53
  Top 0.254: D26.CKI 24.32,19.53 24.85,19 24.85,9.77 24.32,9.24 D25.CKO
N$54
  Top 0.254: D26.SDI D25.SDO
N$55
  Top 0.254: D27.CKI D26.CKO
N$56
  Top 0.254: D27.SDI 22.72,28.42 22.19,27.89 22.19,18.66 22.72,18.13 D26.SDO
N$57
  Top 0.254: D28.CKI 24.32,37.31 24.85,36.78 24.85,27.55 24.32,27.02 D27.CKO
N$58
  Top 0.254: D28.SDI D27.SDO
N$59
  Top 0.254: D29.CKI D28.CKO
N$60
  Top 0.254: D29.SDI 22.72,46.2 22.19,45.67 22.19,36.44 22.72,35.91 D28.SDO
N$61
  Top 0.254: D30.CKI 24.32,55.09 24.85,54.56 24.85,45.33 24.32,44.8 D29.CKO
N$62
  Top 0.254: D30.SDI D29.SDO
N$63
  Top 0.254: D31.CKI D30.CKO
N$64
  Top 0.254: D31.SDI 22.72,63.98 22.19,63.45 22.19,54.22 22.72,53.69 D30.SDO
N$66
  Top 0.254: D32.CKI 24.32,72.87 24.85,72.34 24.85,63.11 24.32,62.58 D31.CKO
N$67
  Top 0.254: D32.SDI D31.SDO
N$68
  Top 0.254: D33.CKI D32.CKO
N$69
  Top 0.254: D33.SDI 22.72,81.76 22.19,81.23 22.19,72 22.72,71.47 D32.SDO
N$70
  Top 0.254: D34.CKI 24.32,90.65 24.85,90.12 24.85,80.89 24.32,80.36 D33.CKO
N$72
  Top 0.254: D34.SDI D33.SDO
N$73
  Top 0.254: D35.CKI D34.CKO
N$74
  Top 0.254: D35.SDI 22.72,99.54 22.19,99.01 22.19,89.78 22.72,89.25 D34.SDO
N$75
  Top 0.254: D36.CKI 24.35,108.44 24.88,107.91 24.88,98.7 24.32,98.14 D35.CKO
N$77
  Top 0.254: D36.SDI 24.35,99.72 D35.SDO
N$79
  Top 0.254: D37.CKO 32.6,99.72 D38.CKI
N$81
  Top 0.254: D37.SDO 32.6,108.44 33.13,107.91 33.13,98.7 32.57,98.14 D38.SDI
N$82
  Top 0.254: D38.CKO 30.97,99.54 30.44,99.01 30.44,89.78 30.97,89.25 D39.CKI
N$91
  Top 0.254: D38.SDO D39.SDI
N$102
  Top 0.254: D39.CKO D40.CKI
N$103
  Top 0.254: D39.SDO 32.57,90.65 33.1,90.12 33.1,80.89 32.57,80.36 D40.SDI
N$104
  Top 0.254: D40.CKO 30.97,81.76 30.44,81.23 30.44,72 30.97,71.47 D41.CKI
N$105
  Top 0.254: D40.SDO D41.SDI
N$106
  Top 0.254: D41.CKO D42.CKI
N$107
  Top 0.254: D41.SDO 32.57,72.87 33.1,72.34 33.1,63.11 32.57,62.58 D42.SDI
N$108
  Top 0.254: D42.CKO 30.97,63.98 30.44,63.45 30.44,54.22 30.97,53.69 D43.CKI
N$109
  Top 0.254: D42.SDO D43.SDI
N$110
  Top 0.254: D43.CKO D44.CKI
N$111
  Top 0.254: D43.SDO 32.57,55.09 33.1,54.56 33.1,45.33 32.57,44.8 D44.SDI
N$112
  Top 0.254: D44.CKO 30.97,46.2 30.44,45.67 30.44,36.44 30.97,35.91 D45.CKI
N$113
  Top 0.254: D44.SDO D45.SDI
N$114
  Top 0.254: D45.CKO D46.CKI
N$115
  Top 0.254: D45.SDO 32.57,37.31 33.1,36.78 33.1,27.55 32.57,27.02 D46.SDI
N$116
  Top 0.254: D46.CKO 30.97,28.42 30.44,27.89 30.44,18.66 30.97,18.13 D47.CKI
N$117
  Top 0.254: D46.SDO D47.SDI
N$118
  Top 0.254: D47.CKO D48.CKI
N$119
  Top 0.254: D47.SDO 32.57,19.53 33.1,19 33.1,9.77 32.57,9.24 D48.SDI
N$120
  Top 0.254: D50.CKI 40.83,19.53 41.36,19 41.36,9.77 40.83,9.24 D49.CKO
N$121
  Top 0.254: D50.SDI D49.SDO
N$122
  Top 0.254: D51.CKI D50.CKO
N$123
  Top 0.254: D51.SDI 39.23,28.42 38.7,27.89 38.7,18.66 39.23,18.13 D50.SDO
N$124
  Top 0.254: D52.CKI 40.83,37.31 41.36,36.78 41.36,27.55 40.83,27.02 D51.CKO
N$125
  Top 0.254: D52.SDI D51.SDO
N$126
  Top 0.254: D53.CKI D52.CKO
N$127
  Top 0.254: D53.SDI 39.23,46.2 38.7,45.67 38.7,36.44 39.23,35.91 D52.SDO
N$128
  Top 0.254: D54.CKI 40.83,55.09 41.36,54.56 41.36,45.33 40.83,44.8 D53.CKO
N$129
  Top 0.254: D54.SDI D53.SDO
N$130
  Top 0.254: D55.CKI D54.CKO
N$131
  Top 0.254: D55.SDI 39.23,63.98 38.7,63.45 38.7,54.22 39.23,53.69 D54.SDO
N$132
  Top 0.254: D56.CKI 40.83,72.87 41.36,72.34 41.36,63.11 40.83,62.58 D55.CKO
N$133
  Top 0.254: D56.SDI D55.SDO
N$134
  Top 0.254: D58.CKI 40.83,90.65 41.36,90.12 41.36,80.89 40.83,80.36 D57.CKO
N$135
  Top 0.254: D58.SDI D57.SDO
N$136
  Top 0.254: D59.CKI D58.CKO
N$137
  Top 0.254: D59.SDI 39.23,99.54 38.7,99.01 38.7,89.78 39.23,89.25 D58.SDO
N$138
  Top 0.254: D60.CKI 40.85,108.44 41.38,107.91 41.38,98.69 40.83,98.14 D59.CKO
N$139
  Top 0.254: D60.SDI 40.85,99.71 D59.SDO
N$140
  Top 0.254: D57.CKI D56.CKO
N$141
  Top 0.254: D57.SDI 39.23,81.76 38.7,81.23 38.7,72 39.23,71.47 D56.SDO
N$157
  Bottom 0.203: R2.1 5.65,27.74 6.05,28.14 6.05,29.34 6.3,29.59 U1.2
N$158
  Bottom 0.203: U1.3 6.1,30.09 5.43,29.42 5.43,28.77 5.21,28.54 3.45,28.54 3.35,28.64 R3.2
N$159
  Bottom 0.203: R3.1 C64.1 4.9,30.59 U1.4
N$162
  Bottom 0.203: R4.1 R5.2 5.3,31.59 U1.6
SD  (via drill 0.35)
  Top 0.254: D1.SDI 11.32,5.58 v27.43,5.58
  Bottom 0.254: Q3.3 30.5,12.39 R10.2 28.88,12.46 28.26,12.46 27.43,11.63 v27.43,5.58
SD1
  Top 0.254: D12.SDO D13.SDI
SD2
  Top 0.254: D25.SDI 22.72,10.64 19.69,7.61 14.82,7.61 14.46,7.96 D24.SDO
SD3
  Top 0.254: D36.SDO 22.75,107.04 22.22,107.57 22.22,110.08 22.8,110.66 29.08,110.66 31,108.74 D37.SDI
SD4
  Top 0.254: D49.SDI 39.23,10.49 36.35,7.61 30.87,7.61 30.63,7.85 30.63,8.75 D48.SDO
SW1
  Bottom 0.305: U1.10 9.95,29.84
  pour Bottom (isolate 0.203, no thermals): 9.85,29.94 15.35,29.94 15.35,27.74 11.45,27.74 9.95,29.04 9.95,29.84
SW2
  Bottom 0.254: U1.8 10.55,30.84 10.75,31.04 11.5,31.04 L1.2
  pour Bottom (isolate 0.203, no thermals): 9.55,30.94 9.85,30.94 10.05,31.14 10.05,31.64 11.53,33.04 15.25,33.04 15.35,32.94 15.35,30.74 9.55,30.74
VBAT  (via drill 0.3)
  Top 0.203: v3.31,27.72 3.31,21.98 4.25,21.04 v5.75,21.04
  Bottom 0.203: R2.2 3.33,27.74 v3.31,27.72 | 9.65,28.54 9.55,28.44 C63.1 | v5.75,21.04 5.75,20.3 WIPHONE_DAUGHTERBOARD-FOOTPRINT1.12
  Bottom 1.778: WIPHONE_DAUGHTERBOARD-FOOTPRINT1.12 10.43,24.54
  pour Bottom (isolate 0.203, rank 2, no thermals): 8.75,29.44 8.75,27.04 9.05,26.74 9.05,24.04 9.15,23.94 12.45,23.94 12.45,27.04 12.15,27.34 11.25,27.34 9.65,28.94 9.65,29.44
VCC  (via drill 0.3, 0.5)
  Top 0.254: D11.VDD C50.2 9.01,100.78 9.35,100.74 | D10.VDD C51.2 7.06,87.84 9.35,87.84 | D9.VDD C52.2 7.07,83.24 9.35,83.24 | D8.VDD C53.2 7.08,70.24 9.35,70.24 | D7.VDD C54.2 7.09,65.34 9.35,65.34 | D6.VDD C55.2 9.04,52.35 9.35,52.34 | D5.VDD C56.2 9.05,47.54 9.35,47.54 | D1.VDD C60.2 7.07,12.04 10.35,12.04 | 10.35,16.54 10.08,16.81 C59.2 D2.VDD | 10.35,29.64 10.15,29.64 7.13,29.64 C58.2 D3.VDD | 9.35,105.64 8.98,105.71 C49.2 7.05,105.75 D12.VDD | 13.15,12.14 13.19,12.18 C37.1 15.25,10.66 D24.VDD | 13.15,16.84 13.18,16.81 C38.1 15.26,16.82 D23.VDD | 13.15,29.84 15.23,29.84 C39.1 15.25,28.44 D22.VDD | 13.15,34.54 13.24,34.63 C40.1 15.26,34.64 D21.VDD | 13.15,47.64 15.21,47.64 C41.2 15.3,47.63 D20.VDD | 13.15,52.14 15.04,52.14 C42.2 15.26,52.36 D19.VDD | 13.15,65.54 15.23,65.54 C43.2 15.25,64 D18.VDD | D17.VDD 15.26,70.18 C44.2 15.12,70.04 13.15,70.04 | 13.15,83.24 13.19,83.2 C45.2 15.25,81.78 D16.VDD | 13.15,87.84 13.2,87.89 C46.2 15.26,87.9 D15.VDD | 13.15,100.84 13.19,100.88 C47.2 15.25,99.56 D14.VDD | 13.15,105.74 13.22,105.81 C48.2 15.3,105.86 D13.VDD | D25.VDD 23.52,8.03 C36.1 25.41,8 25.85,8.14 | 25.85,21.24 23.72,21.24 C35.1 23.52,21.04 D26.VDD | 25.85,25.54 23.67,25.54 C34.1 23.55,26.99 D27.VDD | 25.85,38.84 25.54,38.83 C33.1 23.52,38.8 D28.VDD | 25.85,43.44 23.63,43.44 C32.1 23.55,44.77 D29.VDD | D31.VDD 23.52,61.19 C30.1 25.43,61.16 25.85,61.04 | 25.85,56.44 25.46,56.53 C31.1 23.52,56.5 D30.VDD | D32.VDD 23.52,74.68 C29.1 23.62,74.64 25.85,74.64 | 25.85,78.94 23.61,78.94 C28.1 23.52,78.91 D33.VDD | 25.85,92.04 25.5,91.99 C27.1 23.52,91.96 D34.VDD | D35.VDD 23.52,96.73 C26.1 25.49,96.7 25.85,96.64
  Top 0.254: D36.VDD 23.55,109.44 23.75,109.64 25.25,109.64 25.58,109.31 C25.1 25.58,105.87 25.85,105.84 | v28.15,10.14 28.15,10.94 29.55,12.34 31.62,12.34 C13.1 31.75,10.67 D48.VDD | D47.VDD 31.77,16.53 C14.1 29.62,16.51 29.55,16.44 | D46.VDD 31.77,30.24 C15.1 31.63,30.14 29.55,30.14 | 29.55,52.14 29.64,52.05 C18.1 31.77,52.07 D43.VDD | 29.55,47.94 29.57,47.92 C17.1 31.75,46.23 D44.VDD | D42.VDD 31.77,65.5 C19.1 29.67,65.52 29.55,65.64 | 29.55,69.94 29.58,69.97 C20.1 31.77,69.99 D41.VDD | D40.VDD 31.77,83.28 C21.1 29.69,83.3 29.55,83.44 | 29.55,87.24 31.7,87.24 C22.1 31.77,87.31 D39.VDD | 29.55,105.44 29.62,105.51 C24.1 31.8,105.56 D37.VDD | 29.55,100.74 29.69,100.88 C23.1 31.77,100.76 D38.VDD | C1.1 | C1.1 D60.VDD | 42.15,108.54 40.85,109.84 40.06,109.84 C1.1 | 42.15,96.44 41.99,96.6 C2.1 40.05,98.12 D59.VDD | 42.15,92.64 42.1,92.59 C3.1 40.03,92.57 D58.VDD | D57.VDD 40.03,78.8 C4.1 42.01,78.78 42.15,78.64 | 42.15,74.74 42.12,74.71 C5.1 40.03,74.69 D56.VDD | D55.VDD 40.03,61.28 C6.1 42.07,61.26 42.15,61.34 | 42.15,56.84 C7.1 40.03,56.81 D54.VDD | D53.VDD 40.03,43.46 C8.1 40.45,43.44 40.95,42.94 40.95,39.54 41.54,38.95 | D52.VDD 40.03,38.93 C9.1 41.54,38.95 | D51.VDD 40.03,25.34 C10.1 40.07,25.34 42.15,25.34 | C11.1 40.08,21.24 | 40.08,21.24 42.15,21.24 | D49.VDD 40.03,7.46 C12.1 40.85,7.44 42.15,8.74 42.15,12.44 | 41.54,38.95 41.55,38.94 | D45.VDD 31.77,33.98 C16.1 29.64,33.96 29.55,34.04 | 9.69,35.77 9.69,35.72 C57.2 7.15,35.03 7.01,35.16 D4.VDD 7.01,36.33 v6.8,36.54 | D50.VDD 40.03,21.19 40.08,21.24
  Top 0.508: 10.15,34.94 10.15,35.14 | v42.15,31.14 42.15,38.34 41.55,38.94
  Top 0.813: 13.15,12.14 13.15,16.84 13.15,29.84 13.15,34.54 v13.15,35.54 13.15,47.64 13.15,52.14 13.15,65.54 13.15,70.04 13.15,83.24 13.15,87.84 13.15,100.84 13.15,105.74 | 10.35,12.04 10.35,16.54 10.35,29.64 | 10.15,29.64 v10.15,34.34 10.15,34.94 | 10.15,35.14 9.69,35.77 9.35,36.24 9.35,47.54 9.35,52.34 9.35,65.34 9.35,70.24 9.35,83.24 9.35,87.84 9.35,100.74 9.35,105.64 | 29.55,12.34 29.55,16.44 29.55,30.14 29.55,34.04 v29.55,35.84 29.55,47.94 29.55,52.14 29.55,65.64 29.55,69.94 29.55,83.44 29.55,87.24 29.55,100.74 29.55,105.44 | 25.85,8.14 25.85,21.24 25.85,25.54 v25.85,35.34 v25.85,35.84 | v25.85,35.84 25.85,38.84 25.85,43.44 25.85,56.44 25.85,61.04 25.85,74.64 25.85,78.94 25.85,92.04 25.85,96.64 25.85,105.84 | 42.15,12.44 42.15,21.24 42.15,25.34 v42.15,31.14 | v42.15,51.64 42.15,56.84 42.15,61.34 42.15,74.74 42.15,78.64 42.15,92.64 42.15,96.44 42.15,108.54 | v25.85,36.34 v25.85,35.84
  Bottom 0.254: v28.15,10.14 28.7,10.69 R10.1 R7.1 | R4.2 3.35,34.94 5.05,36.64 6.7,36.64 v6.8,36.54
  Bottom 0.813: v42.15,51.64 37.75,51.64 35.95,49.84 v35.95,35.94 v35.95,35.24 v35.95,34.54 35.95,32.34 37.15,31.14 v42.15,31.14 | C62.1 v10.15,34.34
  other vias: 13.15,34.94 13.15,34.34 29.55,35.24 29.55,34.64 9.65,35.84
  pour Bottom (isolate 0.203, rank 2, no thermals): 8.75,31.54 8.75,36.54 9.05,36.84 37.05,36.84 37.05,33.34 11.35,33.34 9.55,31.54

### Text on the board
bPlace: v2.1
bNames: GND | VBAT | GND | GND | 3.3V | EN | DATA | CLK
